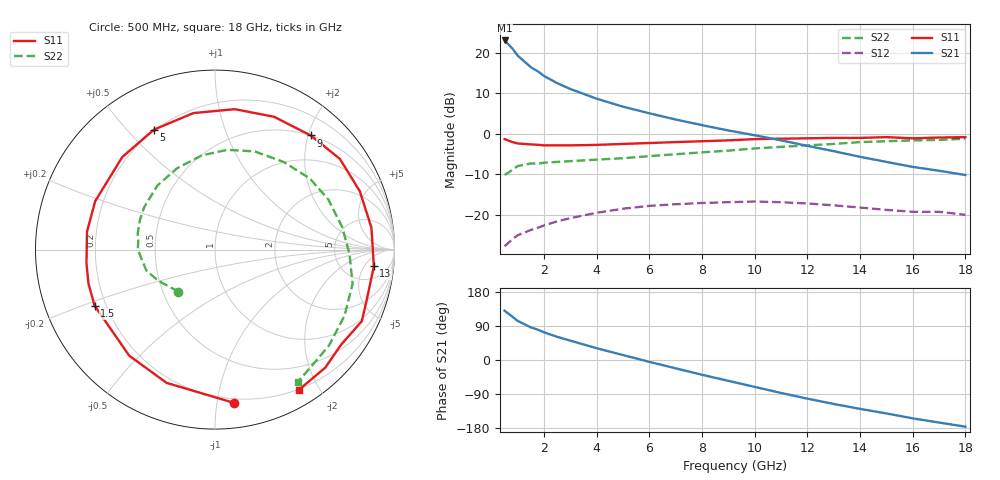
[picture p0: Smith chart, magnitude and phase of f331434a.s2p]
!ATF-33143
!S-PARAMETERS at Vds=4V  Id=60mA.  LAST UPDATED 09-29-99
# ghz s ma r 50
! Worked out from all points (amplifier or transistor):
!   23 points, 500 MHz to 18 GHz, reference 50 ohm
!   highest |S21| = 23.1 dB at 500 MHz (marker M1)
!   |S21| within 3 dB of that: start of sweep to 911.8 MHz
!   unconditionally stable (mu >= 1): 3.785 GHz to end of sweep
!   at 1.5 GHz: K = 0.66, MSG = 20.1 dB, |S12| = -23.7 dB
!   at 7 GHz: K = 1.11, MAG = 8.4 dB, |S12| = -17.4 dB
!   at 18 GHz: K = 1.41, MAG = 1.1 dB, |S12| = -20.0 dB
!   lowest NFmin = 0.11 dB at 500 MHz
!   S11 on the Smith chart (normalised r, x): 500 MHz: 0.17, -1.12; 1.5 GHz: 0.16, -0.22; 5 GHz: 0.20, +0.60; 9 GHz: 0.50, +2.04; 13 GHz: 10, -9; 18 GHz: 0.19, -1.75
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0.5  0.86 -83.0  14.21 130.0  0.041 51.0  0.31 -131.0
0.8  0.79 -110.0  11.25 114.0  0.05 43.0  0.36 -151.0
1  0.76 -129.0  9.21 103.0  0.056 38.0  0.4 -163.0
1.5  0.74 -155.0  6.63 86.0  0.065 32.0  0.43 -180.0
1.8  0.73 -165.0  5.8 79.0  0.07 30.0  0.43 174.0
2  0.72 -174.0  5.16 73.0  0.074 28.0  0.44 168.0
2.5  0.72 172.0  4.22 61.0  0.083 24.0  0.45 158.0
3  0.72 158.0  3.57 51.0  0.091 20.0  0.46 149.0
4  0.73 135.0  2.71 31.0  0.106 11.0  0.48 132.0
5  0.75 117.0  2.16 13.0  0.119 0.0  0.5 115.0
6  0.77 99.0  1.79 -5.0  0.129 -12.0  0.53 98.0
7  0.79 82.0  1.5 -22.0  0.135 -25.0  0.56 83.0
8  0.81 66.0  1.28 -39.0  0.14 -37.0  0.59 68.0
9  0.83 50.0  1.1 -55.0  0.143 -49.0  0.62 52.0
10  0.86 36.0  0.96 -71.0  0.146 -62.0  0.66 37.0
11  0.87 22.0  0.83 -87.0  0.143 -75.0  0.69 24.0
12  0.88 8.0  0.71 -102.0  0.138 -87.0  0.72 10.0
13  0.89 -6.0  0.61 -116.0  0.131 -98.0  0.75 -2.0
14  0.89 -18.0  0.52 -129.0  0.123 -108.0  0.79 -14.0
15  0.91 -26.0  0.45 -141.0  0.115 -117.0  0.81 -27.0
16  0.88 -37.0  0.39 -154.0  0.109 -127.0  0.83 -40.0
18  0.91 -59.0  0.31 -176.0  0.1 -145.0  0.87 -58.0
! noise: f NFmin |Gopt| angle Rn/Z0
0.5  0.11  0.72  38  0.07
0.9  0.15  0.66  58  0.07
1.5  0.22  0.57  86  0.05
1.8  0.26  0.52  101  0.05
2.5  0.35  0.43  133  0.03
3  0.42  0.4  154  0.03
5  0.7  0.42  -140  0.06
6  0.84  0.49  -114  0.12
8  1.12  0.64  -74  0.38
10  1.4  0.65  -41  0.82
